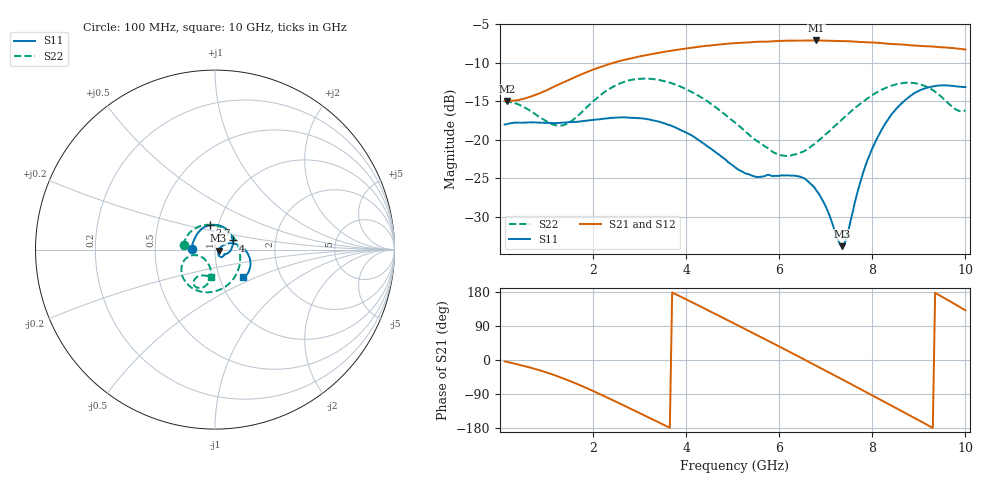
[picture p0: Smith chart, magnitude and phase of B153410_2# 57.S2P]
!  2-Port S-parameters saved by WinCal
! VAR MeasName=S-Parameters (CALIBRATED_DATA) read from VNA (N5245A)
! VAR MeasDate=2016-12-23 10:02:25
! VAR NAME=B153410_2# 57
! VAR FILENAME=B153410_2# 57.S2P
! VAR DATE=2016-12-23 10:02:25
! VAR PHYS_PORTS=1,2
# Hz S DB R 50
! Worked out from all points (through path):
!   199 points, 100 MHz to 10 GHz, reference 50 ohm
!   highest |S21| = -7.11 dB at 6.8 GHz (marker M1); lowest = -15.0 dB at 150 MHz (marker M2)
!   lowest |S11| = -33.9 dB at 7.35 GHz (marker M3), VSWR 1.04, Z = 52 - j0.548 ohm
!   |S11| at or under -10 dB: start of sweep to end of sweep
!   |S22| runs from -22.1 to -12.1 dB; largest |S21 - S12| = 0.004
!   S11 on the Smith chart (normalised r, x): 100 MHz: 0.78, +0.00; 2.7 GHz: 0.91, +0.25; 4 GHz: 1.21, +0.12; 10 GHz: 1.30, -0.42
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1e8  -18.03 179.4  -14.96 -3.7  -14.96 -3.7  -15.06 172.3
1.5e8  -18.00 178.3  -14.99 -5.1  -14.96 -5.3  -15.06 168.1
9.5e8  -17.81 159.0  -13.71 -30.8  -13.72 -30.8  -17.43 86.9
1.35e9  -17.80 149.8  -12.60 -48.1  -12.59 -48.2  -18.14 31.6
1.75e9  -17.61 139.3  -11.51 -68.2  -11.52 -68.2  -16.48 -20.6
2.7e9  -17.10 102.4  -9.59 -122.3  -9.61 -122.2  -12.43 -96.8
3.4e9  -17.63 63.9  -8.73 -163.8  -8.74 -163.8  -12.22 -131.0
4e9  -19.07 27.2  -8.15 160.0  -8.15 160.1  -13.42 -151.4
4.45e9  -20.85 1.6  -7.79 132.4  -7.80 132.6  -14.99 -161.5
5.05e9  -23.58 -21.9  -7.45 95.2  -7.46 95.4  -17.77 -165.9
5.8e9  -24.62 -32.2  -7.25 48.2  -7.24 48.4  -21.32 -151.4
6.25e9  -24.68 -40.2  -7.13 19.8  -7.14 19.8  -22.07 -131.7
6.7e9  -25.89 -52.8  -7.11 -9.0  -7.12 -9.0  -20.81 -112.3
6.8e9  -26.62 -55.5  -7.11 -15.4  -7.12 -15.3  -20.37 -109.2
7.35e9  -33.85 -15.0  -7.19 -50.9  -7.18 -50.9  -17.37 -99.2
7.45e9  -32.67 7.0  -7.20 -57.5  -7.22 -57.4  -16.82 -98.8
7.85e9  -23.44 27.4  -7.34 -83.5  -7.34 -83.4  -14.85 -100.2
8.35e9  -17.28 9.9  -7.54 -116.2  -7.55 -115.9  -13.11 -107.6
8.75e9  -14.64 -7.6  -7.68 -142.6  -7.72 -142.2  -12.58 -115.8
9.2e9  -13.21 -26.1  -7.87 -172.5  -7.87 -172.3  -13.21 -123.6
9.6e9  -12.94 -38.7  -8.03 159.8  -8.03 160.3  -15.09 -122.0
1e10  -13.15 -44.0  -8.30 131.0  -8.30 131.3  -16.20 -98.0
